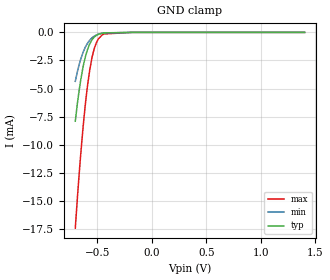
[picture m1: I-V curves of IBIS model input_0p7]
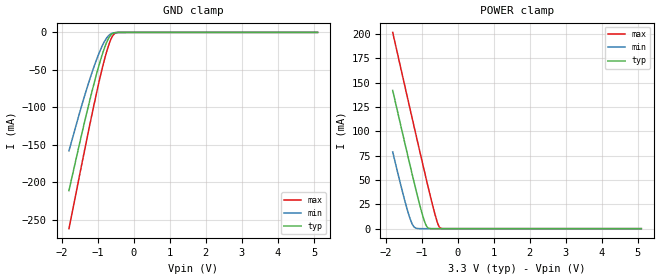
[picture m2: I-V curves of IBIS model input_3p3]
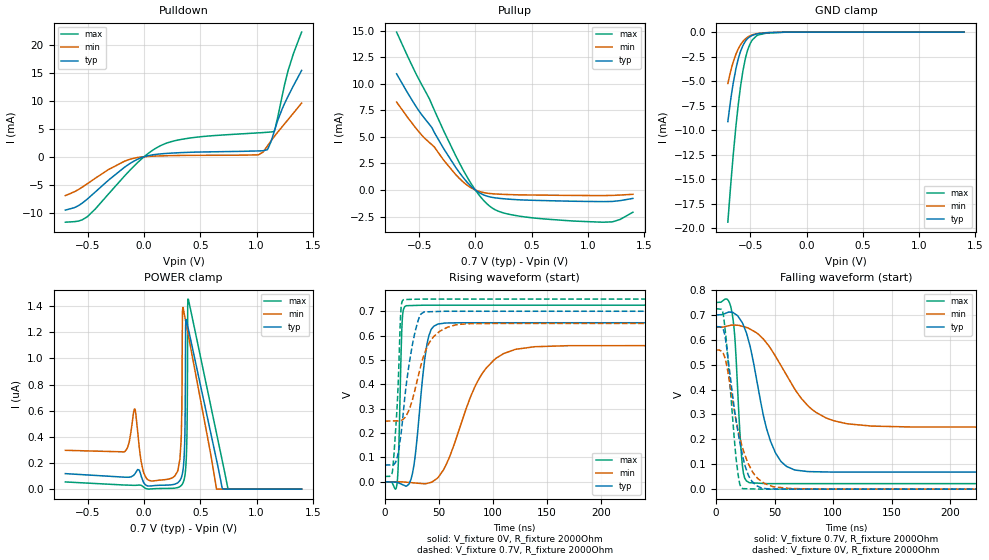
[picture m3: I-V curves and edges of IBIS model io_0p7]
|Texas Instruments Incorporated
|SN74AXC4T245, Quad-Bit Bus Transceiver with Configurable Voltage Translation
|and 3-State Outputs
[IBIS Ver]   4.1
[File name]   sn74axc4t245.ibs
[Date]   12/03/2018
[File Rev]   1.0
[Source]
| Texas Instruments Incorporated.
| Analog-eLab Design Center, HPA
| 12500 TI Blvd
| Dallas, TX -75243
[Notes]   Revision History:
| Rev 1.0: 12/03/2018
| - Initial version of the model
| - Model generated from simulations in SPECTRE
| - Model names with a trailing _0p7 contain the model for 0.7V operation.
|   Model names with a trailing _3p3 contain the model for 3.3V operation.
| - C_comp although listed in numerical order of value are
|   obtained from varying PVT conditions. For PVT conditions for
|   each specific value refer the buffer description under
|   respective [Model]. IBIS model user is responsible for using
|   appropriate C_comp to simulate for Signal Integrity.
[Disclaimer]
| This model is designed as an aid for customers of Texas Instruments.
| TI and its licensors and suppliers make no warranties, either expressed
| or implied, with respect to this  model, including the warranties of
| merchantability or fitness for a particular purpose. The model is
| provided solely on an "as is" basis. The entire risk as to its quality
| and performance is with the customer.
| This model is subject to change without notice. Texas Instruments
| Incorporated is not responsible for updating this model.
[Copyright]
(C) Copyright 2018 Texas Instruments Incorporated.All rights reserved.
|  Component SN74AXC4T245BQB 16-Pin VQFN -BQB package
|  Part # SN74AXC4T245BQB
[Component]   SN74AXC4T245BQB
[Manufacturer]  TI
[Package]   |16 VQFN - BQB package
|   typ   min   max
R_pkg   0.05   0.04   0.06
L_pkg   1.0nH   0.8nH   1.2nH
C_pkg   0.2pF   0.16pF   0.24pF
[Pin]  signal_name  model_name  R_pin   L_pin   C_pin
1   VCCA   power   NA   NA   NA
2   1DIR   input   NA   NA   NA
3   2DIR   input   NA   NA   NA
4   1A1   io   NA   NA   NA
5   1A2   io   NA   NA   NA
6   2A1   io   NA   NA   NA
7   2A2   io   NA   NA   NA
8   GND   gnd   NA   NA   NA
9   GND   gnd   NA   NA   NA
10   2B2   io   NA   NA   NA
11   2B1   io   NA   NA   NA
12   1B2   io   NA   NA   NA
13   1B1   io   NA   NA   NA
14   2OEb   input   NA   NA   NA
15   1OEb   input   NA   NA   NA
16   VCCB   power   NA   NA   NA
|  Component SN74AXC4T245PW 16-Pin TSSOP -PW package
|  Part # SN74AXC4T245PW
[Component]   SN74AXC4T245PW
[Manufacturer]  TI
[Package]   |16 TSSOP - PW package
|   typ   min   max
R_pkg   0.05   0.04   0.06
L_pkg   1.0nH   0.8nH   1.2nH
C_pkg   0.2pF   0.16pF   0.24pF
[Pin]  signal_name  model_name  R_pin   L_pin   C_pin
1   VCCA   power   NA   NA   NA
2   1DIR   input   NA   NA   NA
3   2DIR   input   NA   NA   NA
4   1A1   io   NA   NA   NA
5   1A2   io   NA   NA   NA
6   2A1   io   NA   NA   NA
7   2A2   io   NA   NA   NA
8   GND   gnd   NA   NA   NA
9   GND   gnd   NA   NA   NA
10   2B2   io   NA   NA   NA
11   2B1   io   NA   NA   NA
12   1B2   io   NA   NA   NA
13   1B1   io   NA   NA   NA
14   2OEb   input   NA   NA   NA
15   1OEb   input   NA   NA   NA
16   VCCB   power   NA   NA   NA
|  Component SN74AXC4T245RSV 16-Pin UQFN -RSV package
|  Part # SN74AXC4T245RSV
[Component]   SN74AXC4T245RSV
[Manufacturer]  TI
[Package]   |16 UQFN - RSV package
|   typ   min   max
R_pkg   0.05   0.04   0.06
L_pkg   1.0nH   0.8nH   1.2nH
C_pkg   0.2pF   0.16pF   0.24pF
[Pin]  signal_name  model_name  R_pin   L_pin   C_pin
1   1OEb   input   NA   NA   NA
2   VCCB   power   NA   NA   NA
3   VCCA   power   NA   NA   NA
4   1DIR   input   NA   NA   NA
5   2DIR   input   NA   NA   NA
6   1A1   io   NA   NA   NA
7   1A2   io   NA   NA   NA
8   2A1   io   NA   NA   NA
9   2A2   io   NA   NA   NA
10   GND   gnd   NA   NA   NA
11   GND   gnd   NA   NA   NA
12   2B2   io   NA   NA   NA
13   2B1   io   NA   NA   NA
14   1B2   io   NA   NA   NA
15   1B1   io   NA   NA   NA
16   2OEb   input   NA   NA   NA
|   Model Selectors
[Model Selector] input
input_0p7   0.7V   digital Input
input_3p3   3.3V   digital Input
[Model Selector] io
io_0p7   0.7V   digital I/O
io_3p3   3.3V   digital I/O
| Models and submodels in the file (4): input_0p7 (Input), input_3p3 (Input), io_0p7 (I/O), io_3p3 (I/O)
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|   input_0p7 Model
[Model]   input_0p7
Model_type   Input
Vinl = 0.21
Vinh = 0.49
|   typ   min   max
C_comp   7.40696E-13   6.45127E-13   8.98734E-13
[Model spec]
|subparameter
Vinl   0.21   0.195   0.225
Vinh   0.49   0.455   0.525
| Where Nom  PVT is Nominal Process, 0.7V, 27C
|   Fast PVT is Strong Process,  0.75V, -40C
|   Slow PVT is Weak Process,   0.65, 130C
[Voltage Range]   0.7   0.65   0.75
|Junction Temperature
[Temperature Range]   27   130   -40
[Power Clamp Reference]   0.7   0.65   0.75
[GND Clamp Reference]   0   0   0
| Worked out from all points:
|   GND clamp passes 1 mA (typ) near -0.57 V on its own axis
[GND Clamp]
|   Voltage   I(typ)   I(min)   I(max)
-700mV    -7.896mA   -4.354mA   -17.4mA
-676.9mV  -6.033mA   -3.335mA   -14.2mA
-651.7mV  -4.329mA   -2.43mA    -11.02mA
-624.4mV  -2.873mA   -1.673mA   -7.992mA
-588.7mV  -1.545mA   -978.4uA   -4.797mA
-567.7mV  -1.026mA   -696.2uA   -3.358mA
-548.8mV  -691.6uA   -504.6uA   -2.342mA
-527.8mV  -434.7uA   -346.8uA   -1.503mA
-487.9mV  -168.3uA   -161.7uA   -574.9uA
-454.3mV  -71.1uA    -80.61uA   -230.7uA
-175mV    -4.456nA   -77.57nA   0A
1.4V      0A         0A         0A
[POWER Clamp]
|   Voltage   I(typ)   I(min)   I(max)
-700mV    0A         0A         0A
0V        0A         0A         0A
1.4V      0A         0A         0A
|   input_3p3 Model
[Model]   input_3p3
Model_type   Input
Vinl = 0.8
Vinh = 2.0
|   typ   min   max
C_comp   1.86062E-12   1.26954E-12   2.13619E-12
| Where Nom  PVT is Nominal Process, 3.3V, 27C
|   Fast PVT is Strong Process,  3.6V, -40C
|   Slow PVT is Weak Process,   3.0V, 130C
[Voltage Range]   3.3   3   3.6
|Junction Temperature
[Temperature Range]   27   130   -40
[Power Clamp Reference]   3.3   3   3.6
[GND Clamp Reference]   0   0   0
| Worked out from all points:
|   GND clamp passes 1 mA (typ) near -0.57 V on its own axis
|   POWER clamp passes 1 mA (typ) near -0.83 V on its own axis
[GND Clamp]
|   Voltage   I(typ)   I(min)   I(max)
-1.8V     -210.9mA   -157.9mA   -261.6mA
-1.49V    -144.7mA   -104.6mA   -186.5mA
-1.296V   -105.2mA   -73.69mA   -140.6mA
-1.117V   -70.54mA   -47.4mA    -99.2mA
-951.3mV  -41.37mA   -26.15mA   -63.06mA
-820.2mV  -21.52mA   -12.61mA   -37.23mA
-716.7mV  -9.415mA   -5.207mA   -19.86mA
-613.2mV  -2.39mA    -1.422mA   -6.892mA
-523.5mV  -394uA     -320.5uA   -1.365mA
-426.9mV  -33.77uA   -44.18uA   -102.3uA
-68.1mV   0A         0A         0A
5.1V      0A         0A         0A
[POWER Clamp]
|   Voltage   I(typ)   I(min)   I(max)
-1.8V     141.9mA    78.74mA    201.4mA
-1.414V   79.93mA    21.78mA    138.3mA
-1.296V   61.5mA     8.016mA    119.2mA
-1.234V   51.89mA    3.123mA    109.2mA
-1.151V   39.29mA    456.6uA    95.81mA
-985.8mV  15.65mA    4.189uA    69.3mA
-868.5mV  3.093mA    131.9nA    50.79mA
-799.5mV  400.9uA    7.757nA    40.08mA
-571.8mV  47.54nA    0A         7.669mA
-516.6mV  0A         0A         2.383mA
-468.3mV  0A         0A         390.4uA
5.1V      0A         0A         0A
|   io_0p7 Model
[Model]   io_0p7
Model_type   I/O
Polarity   Non-Inverting
Enable   Active-High
Vinl = 0.21
Vinh = 0.49
Vmeas = 0.35
Vref = 0
Cref = 2pF
Rref = 100000
|   typ   min   max
C_comp   1.54049E-12   1.37923E-12   1.78504E-12
[Model spec]
|subparameter
Vinl   0.21   0.195   0.225
Vinh   0.49   0.455   0.525
| Where Nom  PVT is Nominal Process, 0.7V, 27C
|   Fast PVT is Strong Process,  0.75V, -40C
|   Slow PVT is Weak Process,   0.65, 130C
[Voltage Range]   0.7   0.65   0.75
|Junction Temperature
[Temperature Range]   27   130   -40
[Pullup Reference]   0.7   0.65   0.75
[Pulldown Reference]   0   0   0
[Power Clamp Reference]   0.7   0.65   0.75
[GND Clamp Reference]   0   0   0
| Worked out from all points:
|   slope of the pulldown table from 0 to 0.105 V, typ, clamps not added: 251 ohm
|   slope of the pullup table from 0 to 0.105 V, typ, clamps not added: 180 ohm
|   GND clamp passes 1 mA (typ) near -0.55 V on its own axis
|   falling waveform, V_fixture 0.7V, R_fixture 2000Ohm: 20-80 % time 17.3ns typ, 33.8ns min, 5.11ns max; typ from 0.7 V to 0.069 V
|   rising waveform, V_fixture 0V, R_fixture 2000Ohm: 20-80 % time 8.82ns typ, 29.9ns min, 2.41ns max; typ from 0 V to 0.653 V
|   rising waveform, V_fixture 0.7V, R_fixture 2000Ohm: 20-80 % time 11ns typ, 16ns min, 4.59ns max; typ from 0.069 V to 0.7 V
|   falling waveform, V_fixture 0V, R_fixture 2000Ohm: 20-80 % time 12.5ns typ, 15.7ns min, 7.58ns max; typ from 0.653 V to 0 V
[Pulldown]
|   Voltage   I(typ)   I(min)   I(max)
-700mV    -9.53mA    -6.936mA   -11.68mA
-504.7mV  -7.56mA    -4.826mA   -10.71mA
-116.2mV  -1.094mA   -401.5uA   -2.212mA
-700uV    -4.135uA   -1.175uA   -12.02uA
156.8mV   524.2uA    153.9uA    2.074mA
444.5mV   814.4uA    247.4uA    3.433mA
1.016V    1.034mA    340.2uA    4.259mA
1.058V    1.067mA    839.6uA    4.313mA
1.098V    1.317mA    1.959mA    4.368mA
1.156V    4.475mA    3.596mA    4.506mA
1.278V    10.74mA    6.591mA    15.25mA
1.4V      15.4mA     9.579mA    22.24mA
[GND Clamp]
|   Voltage   I(typ)   I(min)   I(max)
-700mV    -9.134mA   -5.242mA   -19.38mA
-664.3mV  -6.083mA   -3.529mA   -14.17mA
-630.7mV  -3.882mA   -2.333mA   -9.91mA
-605.5mV  -2.655mA   -1.67mA    -7.215mA
-567.7mV  -1.415mA   -980.1uA   -4.082mA
-544.6mV  -944.1uA   -698.3uA   -2.722mA
-521.5mV  -629.7uA   -495uA     -1.75mA
-483.7mV  -335.9uA   -282.4uA   -814.3uA
-445.9mV  -193.6uA   -164.6uA   -387.5uA
-351.4mV  -64.76uA   -49.97uA   -92.43uA
-175mV    -4.252uA   -4.028uA   -4.183uA
1.4V      0A         0A         0A
[Pullup]
|   Voltage   I(typ)   I(min)   I(max)
-700mV    10.94mA    8.279mA    14.86mA
-511mV    7.597mA    5.59mA     10.6mA
-385mV    5.85mA     4.251mA    8.008mA
-275.8mV  3.798mA    2.733mA    5.441mA
-116.2mV  1.282mA    830.6uA    2.039mA
-700uV    5.462uA    3.045uA    10.64uA
129.5mV   -653.1uA   -334uA     -1.541mA
213.5mV   -787.5uA   -396.1uA   -2.037mA
360.5mV   -908.5uA   -451.5uA   -2.409mA
881.3mV   -1.064mA   -514.5uA   -2.93mA
1.222V    -1.075mA   -509.2uA   -2.989mA
1.4V      -796uA     -406uA     -2.097mA
[POWER Clamp]
|   Voltage   I(typ)   I(min)   I(max)
-700mV    118.8nA    297.2nA    55.28nA
-82.6mV   116.1nA    614.3nA    29.33nA
18.2mV    29.94nA    86.4nA     4.018nA
255.5mV   34.86nA    88.97nA    6.633nA
318.5mV   66.18nA    231.3nA    19.67nA
337.4mV   106.9nA    801.1nA    35.29nA
341.6mV   123.5nA    1.369uA    41.03nA
360.5mV   347.9nA    1.325uA    93.15nA
379.4mV   1.28uA     1.24uA     350.7nA
389.9mV   1.239uA    1.192uA    1.454uA
744.8mV   0A         0A         6.021nA
1.4V      0A         0A         0A
[Ramp]
R_load = 2000
|   typ   min   max
dV/dt_r   0.391697/8.77565e-09   0.335547/2.98927e-08   0.434999/2.39639e-09
dV/dt_f   0.378832/1.72731e-08   0.240634/3.38318e-08   0.436699/5.08929e-09
[Falling Waveform]
V_fixture = 0.7V
V_fixture_min = 0.65V
V_fixture_max = 0.75V
R_fixture = 2000Ohm
C_fixture = 0F
|   Time   V(typ)   V(min)   V(max)
0s        700mV      650mV      750mV
13.57ns   710.5mV    659mV      711mV
16.42ns   703.2mV    658.6mV    584.9mV
22.45ns   668.6mV    654.1mV    98.27mV
28.31ns   587.6mV    644.9mV    26.3mV
46.67ns   191mV      564.7mV    22.2mV
67.52ns   77.03mV    399.7mV    22.2mV
93.66ns   69.19mV    286.8mV    22.2mV
133.2ns   68.71mV    253.3mV    22.19mV
500ns     68.61mV    248.9mV    22.17mV
[Rising Waveform]
V_fixture = 0V
V_fixture_min = 0V
V_fixture_max = 0V
R_fixture = 2000Ohm
C_fixture = 0F
|   Time   V(typ)   V(min)   V(max)
0s        923.3nV    12.36uV    39.3nV
11.32ns   -1.698mV   -323.5uV   -9.278mV
16.05ns   -11mV      -463.7uV   653.2mV
19.76ns   -18.13mV   -1.707mV   722.7mV
27.05ns   70.28mV    -4.537mV   723.7mV
39.15ns   566mV      -6.545mV   725mV
48.98ns   647.1mV    15.97mV    725mV
87.49ns   652.8mV    425mV      725mV
120.3ns   652.8mV    542.7mV    725mV
500ns     652.8mV    559.3mV    725mV
[Rising Waveform]
V_fixture = 0.7V
V_fixture_min = 0.65V
V_fixture_max = 0.75V
R_fixture = 2000Ohm
C_fixture = 0F
|   Time   V(typ)   V(min)   V(max)
0s        68.61mV    248.9mV    22.17mV
7.377ns   69.87mV    249.7mV    52.86mV
11.84ns   106.3mV    250.2mV    345.4mV
14.84ns   190mV      251mV      699mV
17.61ns   305.8mV    259mV      748.1mV
27.36ns   602mV      367.3mV    749.1mV
36.62ns   697.3mV    524.4mV    750mV
50.9ns    699.3mV    617.7mV    750mV
78.59ns   700mV      648.9mV    750mV
500ns     700mV      650mV      750mV
[Falling Waveform]
|Gnd
V_fixture = 0V
V_fixture_min = 0V
V_fixture_max = 0V
R_fixture = 2000Ohm
C_fixture = 0F
|   Time   V(typ)   V(min)   V(max)
0s        652.8mV    559.3mV    725mV
6.315ns   639.8mV    543.9mV    697.6mV
9.387ns   557.7mV    489.8mV    566.2mV
17.34ns   269.7mV    270.9mV    114.8mV
20.19ns   192.1mV    209.1mV    22.56mV
22.68ns   134.3mV    165.5mV    2.15mV
27.67ns   55.65mV    101.2mV    1.438mV
34.21ns   15.08mV    50.52mV    576.2uV
63.11ns   71.4uV     2.653mV    22.92uV
500ns     923.6nV    12.38uV    138.7nV
